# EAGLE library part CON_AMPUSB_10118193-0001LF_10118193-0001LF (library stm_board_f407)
Micro USB B Type Receptacle
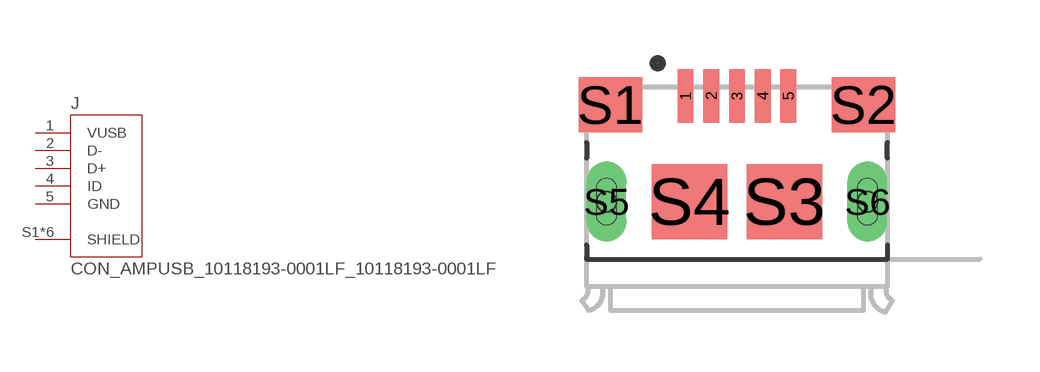
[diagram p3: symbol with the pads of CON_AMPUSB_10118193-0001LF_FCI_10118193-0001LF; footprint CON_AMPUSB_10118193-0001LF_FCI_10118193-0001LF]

Designator prefix J

## CON_AMPUSB_10118193-0001LF_10118193-0001LF (AVAILABILITY: Unavailable; DESCRIPTION: Single Port 5 Contact Shielded SMT MICRO USB B-Type Receptacle; MF: Amphenol ICC; MP: 10118193-0001LF; PACKAGE: None; PRICE: None)  [CON_AMPUSB_10118193-0001LF_FCI_10118193-0001LF]
1  VUSB  pas
2  D-  pas
3  D+  pas
4  ID  pas
5  GND  pas
S1  SHIELD  pas
S2  SHIELD  pas
S3  SHIELD  pas
S4  SHIELD  pas
S5  SHIELD  pas
S6  SHIELD  pas

## Footprint CON_AMPUSB_10118193-0001LF_FCI_10118193-0001LF (pad centres in mm)
smd 0.4 x 1.35: 1 -1.3,2.675; 2 -0.65,2.675; 3 0,2.675; 4 0.65,2.675; 5 1.3,2.675
smd 1.6 x 1.4: S1 -3.2,2.45; S2 3.2,2.45
smd 1.9 x 1.9: S3 1.2,0; S4 -1.2,0
drill 0.5 pad 0.9 long: S5 -3.3,0; S6 3.3,0
hole 0.5 at -3.3,0
hole 0.5 at 3.3,0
